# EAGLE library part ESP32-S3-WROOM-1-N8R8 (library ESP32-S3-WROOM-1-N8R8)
WiFi Modules - 802.11 (Engineering Samples Only) SMD Module, ESP32-S3R8 with 8 MB Octal PSRAM Die, 8 MB Quad SPI flash, PCB Antenna Source: Datasheet
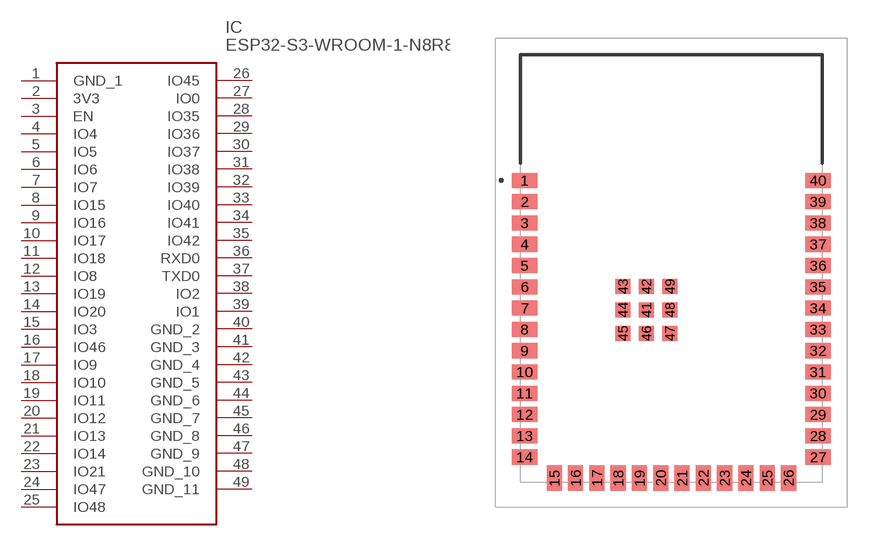
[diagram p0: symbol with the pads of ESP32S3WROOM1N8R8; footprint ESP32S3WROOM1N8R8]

Designator prefix IC

## ESP32-S3-WROOM-1-N8R8 (Description: WiFi Modules - 802.11 (Engineering Samples Only) SMD Module, ESP32-S3R8 with 8 MB Octal PSRAM Die, 8 MB Quad SPI flash, PCB Antenna; Height: 3.25mm; Manufacturer_Name: Espressif Systems; Manufacturer_Part_Number: ESP32-S3-WROOM-1-N8R8; Mouser_Part_Number: 356-EP32S3WROOM1N8R8; Mouser_Price-Stock: https://www.mouser.co.uk/ProductDetail/Espressif-Systems/ESP32-S3-WROOM-1-N8R8?qs=7D1LtPJG0i3%2F28hKFavOpQ%3D%3D)  [ESP32S3WROOM1N8R8]
1  GND_1
2  3V3
3  EN
4  IO4
5  IO5
6  IO6
7  IO7
8  IO15
9  IO16
10  IO17
11  IO18
12  IO8
13  IO19
14  IO20
15  IO3
16  IO46
17  IO9
18  IO10
19  IO11
20  IO12
21  IO13
22  IO14
23  IO21
24  IO47
25  IO48
26  IO45
27  IO0
28  IO35
29  IO36
30  IO37
31  IO38
32  IO39
33  IO40
34  IO41
35  IO42
36  RXD0
37  TXD0
38  IO2
39  IO1
40  GND_2
41  GND_3
42  GND_4
43  GND_5
44  GND_6
45  GND_7
46  GND_8
47  GND_9
48  GND_10
49  GND_11

## Footprint ESP32S3WROOM1N8R8 (pad centres in mm)
ESP32-S3-WROOM-1-N8R8-2
smd 1.5 x 0.9: 1 -8.75,5.26; 2 -8.75,3.99; 3 -8.75,2.72; 4 -8.75,1.45; 5 -8.75,0.18; 6 -8.75,-1.09; 7 -8.75,-2.36; 8 -8.75,-3.63; 9 -8.75,-4.9; 10 -8.75,-6.17; 11 -8.75,-7.44; 12 -8.75,-8.71; 13 -8.75,-9.98; 14 -8.75,-11.25; 27 8.75,-11.25; 28 8.75,-9.98; 29 8.75,-8.71; 30 8.75,-7.44; 31 8.75,-6.17; 32 8.75,-4.9; 33 8.75,-3.63; 34 8.75,-2.36; 35 8.75,-1.09; 36 8.75,0.18; 37 8.75,1.45; 38 8.75,2.72; 39 8.75,3.99; 40 8.75,5.26
smd 0.9 x 1.5: 15 -6.985,-12.5; 16 -5.715,-12.5; 17 -4.445,-12.5; 18 -3.175,-12.5; 19 -1.905,-12.5; 20 -0.635,-12.5; 21 0.635,-12.5; 22 1.905,-12.5; 23 3.175,-12.5; 24 4.445,-12.5; 25 5.715,-12.5; 26 6.985,-12.5
smd 0.9 x 0.9: 41 -1.5,-2.46; 42 -1.5,-1.06; 43 -2.9,-1.06; 44 -2.9,-2.46; 45 -2.9,-3.86; 46 -1.5,-3.86; 47 -0.1,-3.86; 48 -0.1,-2.46; 49 -0.1,-1.06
